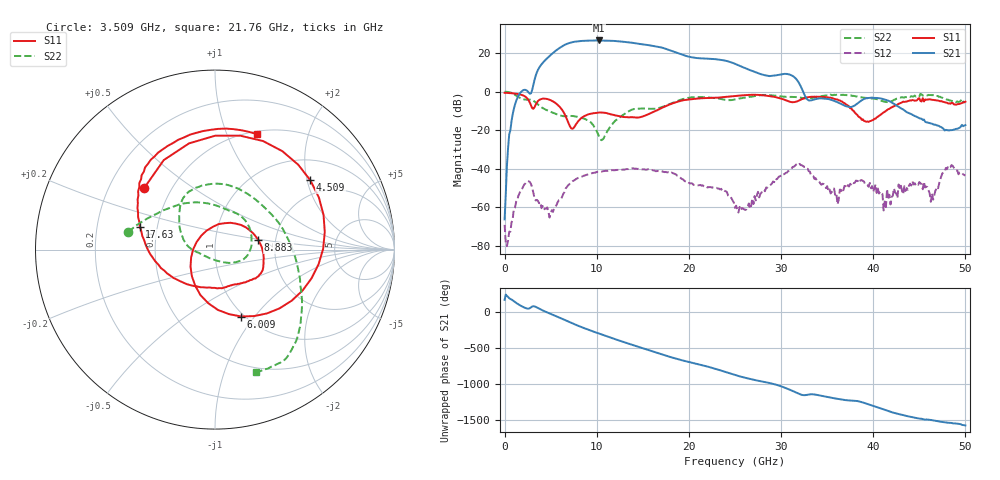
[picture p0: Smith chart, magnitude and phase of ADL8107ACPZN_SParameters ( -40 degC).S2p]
! Analog Devices, Inc.
! Device:	ADL8107ACPZN
! Description:	"GaAs, pHEMT, MMIC, Low Phase Noise Amplifier, 6 GHz to 18 GHz"
! Conditions:	Vdd = 5.0 V
!		IDQ = 90 mA quiescent (Self-biased mode)
!		Pin = -20 dBm
!		Operating Temperature = -40 C (at package bottom)
! Product validation unit SN7 soldered down to Evaluation Board as shown on ADL8107-EVALZ User Guide. Board loss de-embedded from S21 magnitude.  All other RF measurements reference to RF coaxial connector.
! Frequency (GHz)	S11_Mag (dB)	S11_Phase (deg)	S21_Mag (dB)	S21_Phase (deg)	S12_Mag (dB)	S12_Phase (deg)	S22_Mag (dB)	S22_Phase (deg)
#  GHZ  S  DB  R 50
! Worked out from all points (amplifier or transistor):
!   401 points, 10 MHz to 50 GHz, reference 50 ohm
!   highest |S21| = 26.7 dB at 10.26 GHz (marker M1)
!   |S21| within 3 dB of that: 6.266 GHz to 16.35 GHz (10.08 GHz wide, 89.2 % of centre)
!   unconditionally stable (mu >= 1): 62.7 MHz to end of sweep
!   at 8.258 GHz: K = 3.66, MAG = 26.8 dB, |S12| = -44.3 dB
!   at 25.01 GHz: K = 23.38, MAG = 20.8 dB, |S12| = -60.4 dB
!   at 50 GHz: K = 277.18, MAG = -14.3 dB, |S12| = -43.6 dB
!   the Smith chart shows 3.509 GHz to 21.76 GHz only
!   S11 on the Smith chart (normalised r, x): 3.509 GHz: 0.35, +0.33; 4.509 GHz: 1.54, +2.09; 6.009 GHz: 0.97, -0.86; 8.883 GHz: 1.62, +0.18; 17.63 GHz: 0.40, +0.13; 21.76 GHz: 0.53, +1.29
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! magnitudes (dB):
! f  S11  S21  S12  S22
! 10 MHz  -0.6  -66.4  -69.2  0.0
! 509.9 MHz  -0.7  -22.1  -72.7  -0.3
! 1.01 GHz  -0.9  -9.0  -61.0  -1.2
! 2.385 GHz  -3.0  0.8  -46.8  -4.1
! 3.509 GHz  -5.6  10.1  -56.3  -6.2
! 4.509 GHz  -3.7  16.9  -60.8  -9.4
! 6.009 GHz  -7.9  22.9  -56.3  -12.3
! 7.259 GHz  -19.1  25.7  -47.0  -12.6
! 8.383 GHz  -13.5  26.4  -44.2  -13.7
! 8.883 GHz  -12.1  26.6  -43.2  -14.5
! 10.26 GHz  -10.8  26.7  -41.7  -23.3
! 16.76 GHz  -9.1  23.3  -41.3  -8.4
! 17.63 GHz  -7.2  22.1  -41.9  -6.9
! 21.76 GHz  -3.3  17.3  -49.6  -2.9
! 25.01 GHz  -2.2  14.6  -60.4  -4.0
! 31.75 GHz  -5.0  6.0  -37.5  -2.8
! 33.38 GHz  -2.6  -4.3  -43.6  -3.2
! 36.13 GHz  -4.0  -5.4  -58.6  -1.6
! 39.25 GHz  -15.6  -3.3  -48.4  -3.2
! 41.75 GHz  -8.9  -4.9  -53.6  -5.3
! 48.38 GHz  -6.2  -19.9  -39.3  -4.6
! 50 GHz  -5.2  -17.3  -43.6  -5.4
